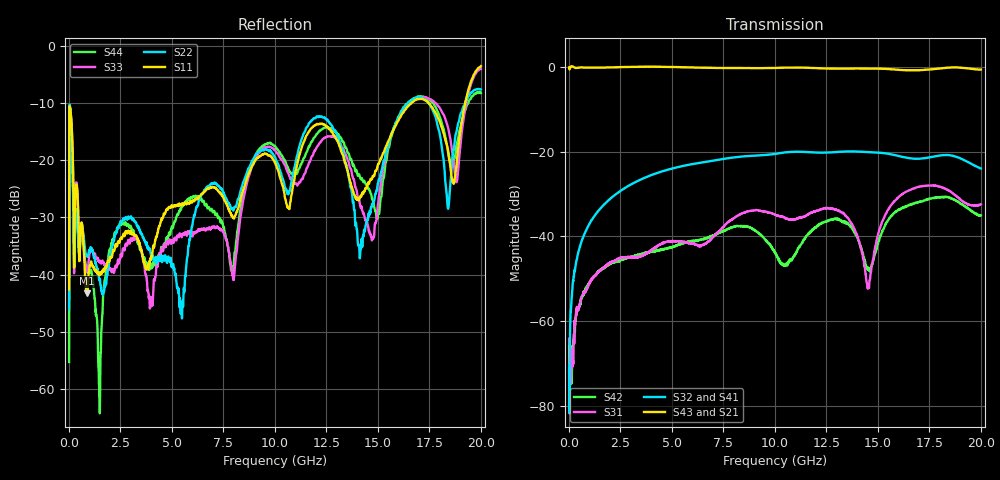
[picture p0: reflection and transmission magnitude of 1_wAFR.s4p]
!Keysight Technologies,N5225A,MY51451420,A.10.40.12
!Date: Tuesday, October 13, 2015 09:32:21
!Correction: S11(Full 4 Port(1,2,3,4))
!S12(Full 4 Port(1,2,3,4))
!S13(Full 4 Port(1,2,3,4))
!S14(Full 4 Port(1,2,3,4))
!S21(Full 4 Port(1,2,3,4))
!S22(Full 4 Port(1,2,3,4))
!S23(Full 4 Port(1,2,3,4))
!S24(Full 4 Port(1,2,3,4))
!S31(Full 4 Port(1,2,3,4))
!S32(Full 4 Port(1,2,3,4))
!S33(Full 4 Port(1,2,3,4))
!S34(Full 4 Port(1,2,3,4))
!S41(Full 4 Port(1,2,3,4))
!S42(Full 4 Port(1,2,3,4))
!S43(Full 4 Port(1,2,3,4))
!S44(Full 4 Port(1,2,3,4))
!S4P File: Measurements: <S11,S12,S13,S14>,
!<S21,S22,S23,S24>,
!<S31,S32,S33,S34>,
!<S41,S42,S43,S44>:
# Hz S  dB  R 50
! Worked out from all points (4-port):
!   2000 points, 10 MHz to 20 GHz, reference 50 ohm
!   strongest paths, dB at 10 MHz, 5.01 GHz, 10.01 GHz, 15.01 GHz, 20 GHz:
!     S43: -0.1, 0.0, -0.2, -0.4, -0.6
!     S21: 0.0, 0.0, -0.2, -0.4, -0.7
!     S32: -71.1, -24.0, -20.5, -20.2, -24.0
!     S41: -64.9, -23.9, -20.6, -20.2, -23.9
!     S31: -64.1, -41.1, -34.9, -39.5, -32.4
!     S42: -72.0, -42.5, -43.9, -41.7, -35.0
!   lowest |S11| = -43.3 dB at 870 MHz (marker M1), VSWR 1.01, Z = 50.6 - j0.365 ohm
!   |S11| at or under -10 dB: start of sweep to 16.64 GHz; 17.46 GHz to 19.24 GHz (1.782 GHz wide, 9.71 % of centre)
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1e7  -42.62 -32.1  -0.02 0.4  -71.37 -25.8  -67.89 95.9
     -0.03 0.5  -46.10 168.5  -71.18 -0.5  -66.55 -133.4
     -64.13 22.4  -71.11 165.1  -40.40 -14.6  -0.06 0.6
     -64.88 95.0  -72.03 -98.5  -0.08 0.1  -55.29 -165.5
1.2e8  -13.15 -107.6  0.16 10.0  -68.36 -11.1  -55.21 94.8
       0.16 10.1  -15.31 -72.8  -55.39 99.3  -68.83 59.6
       -66.73 -19.1  -55.76 97.8  -13.19 -107.7  0.14 10.0
       -54.71 99.3  -71.03 21.4  0.16 10.0  -15.36 -72.6
8.7e8  -43.28 -31.7  -0.15 4.3  -52.50 76.2  -38.21 94.3
       -0.15 4.3  -36.75 14.8  -38.21 93.5  -51.96 111.6
       -52.48 75.8  -38.25 93.7  -39.31 -3.4  -0.17 4.3
       -38.23 94.5  -51.78 111.2  -0.15 4.3  -39.34 36.6
5.46e9  -27.80 -67.5  -0.07 36.2  -41.28 1.6  -23.40 126.9
        -0.08 36.4  -44.98 -53.5  -23.47 124.7  -41.64 -103.1
        -41.32 1.8  -23.46 124.7  -33.23 15.3  -0.07 35.8
        -23.41 127.1  -41.68 -103.2  -0.06 35.8  -28.31 174.5
1.261e10  -14.54 -131.8  -0.46 76.2  -33.35 -72.1  -20.21 168.3
          -0.46 76.6  -13.27 110.4  -20.19 164.1  -36.20 -179.2
          -33.35 -71.7  -20.19 164.0  -15.86 -157.3  -0.40 74.4
          -20.22 168.8  -36.22 -179.6  -0.39 74.5  -14.27 126.2
1.472e10  -23.22 -97.9  -0.42 78.6  -46.56 22.9  -20.12 170.7
          -0.41 79.1  -27.61 64.2  -20.16 165.3  -46.65 -106.2
          -46.58 23.2  -20.16 165.1  -33.77 120.5  -0.39 76.9
          -20.12 171.2  -46.75 -106.1  -0.39 77.1  -26.78 -110.7
2e10  -3.57 -98.3  -0.73 120.5  -32.45 -42.7  -23.93 -150.5
      -0.74 121.1  -7.65 -145.9  -23.95 -156.4  -35.07 -94.3
      -32.44 -42.6  -23.97 -156.9  -4.03 -98.9  -0.63 118.6
      -23.94 -150.1  -35.04 -95.0  -0.62 118.9  -8.27 -144.2
